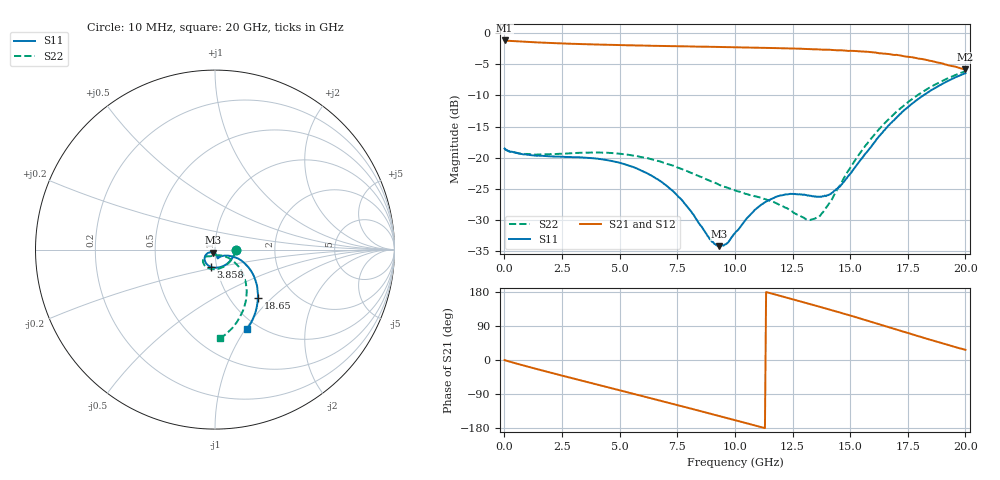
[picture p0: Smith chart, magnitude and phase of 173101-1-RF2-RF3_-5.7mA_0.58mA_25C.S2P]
!  2-Port S-parameters saved by WinCal
! VAR MeasName=S-Parameters (CALIBRATED_DATA) read from VNA (N5242A)
! VAR MeasDate=2017-7-20 9:31:15
! VAR NAME=173101-1-RF2-RF3_-5.7mA_0.58mA_25C
! VAR FILENAME=173101-1-RF2-RF3_-5.7mA_0.58mA_25C.S2P
! VAR DATE=2017-7-20 9:31:15
! VAR PHYS_PORTS=1,2
# Hz S DB R 50
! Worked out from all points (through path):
!   401 points, 10 MHz to 20 GHz, reference 50 ohm
!   highest |S21| = -1.18 dB at 10 MHz (marker M1); lowest = -5.8 dB at 20 GHz (marker M2)
!   group delay of S21, straight-line fit = 45.8 ps
!   lowest |S11| = -34.2 dB at 9.305 GHz (marker M3), VSWR 1.04, Z = 49.1 - j1.73 ohm
!   |S11| at or under -10 dB: start of sweep to 18.17 GHz
!   |S22| runs from -30.0 to -6.1 dB; largest |S21 - S12| = 0.0083
!   S11 on the Smith chart (normalised r, x): 10 MHz: 1.27, -0.00; 3.858 GHz: 0.94, -0.18; 18.65 GHz: 1.34, -0.83; 20 GHz: 0.89, -1.02
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1e7  -18.53 -0.9  -1.18 -0.2  -1.18 -0.3  -18.51 -1.2
1.559225e9  -19.67 -50.8  -1.51 -26.3  -1.51 -26.3  -19.46 -51.2
3.358325e9  -19.96 -92.9  -1.77 -54.5  -1.77 -54.5  -19.20 -91.2
3.858075e9  -20.09 -102.7  -1.82 -62.3  -1.82 -62.2  -19.16 -99.8
5.357325e9  -21.21 -128.6  -1.95 -85.5  -1.97 -85.4  -19.52 -121.7
6.70665e9  -23.60 -146.8  -2.05 -106.6  -2.04 -106.4  -20.54 -135.8
7.70615e9  -26.81 -154.0  -2.12 -122.1  -2.14 -122.0  -21.82 -141.9
8.90555e9  -33.03 -136.4  -2.19 -141.1  -2.20 -140.9  -23.68 -142.8
9.30535e9  -34.19 -115.6  -2.22 -147.5  -2.22 -147.4  -24.32 -141.4
9.6052e9  -33.89 -98.9  -2.24 -152.3  -2.24 -152.1  -24.72 -140.1
1.0005e10  -32.09 -83.0  -2.27 -158.7  -2.28 -158.6  -25.23 -137.2
1.085458e10  -28.40 -70.7  -2.33 -172.4  -2.34 -172.3  -26.17 -130.4
1.145428e10  -26.81 -71.0  -2.38 177.8  -2.38 177.9  -26.81 -125.2
1.230385e10  -25.87 -73.1  -2.45 163.6  -2.46 163.8  -28.20 -114.5
1.335332e10  -26.19 -65.9  -2.58 146.0  -2.57 146.2  -29.88 -81.0
1.375312e10  -26.28 -57.3  -2.64 139.0  -2.64 139.3  -29.01 -61.8
1.455272e10  -24.67 -35.4  -2.74 125.4  -2.74 125.6  -24.47 -36.4
1.575212e10  -18.97 -21.4  -3.01 103.5  -3.02 103.8  -17.67 -33.3
1.670165e10  -14.72 -25.1  -3.37 86.1  -3.42 86.2  -13.72 -41.1
1.76012e10  -11.59 -34.6  -3.83 69.7  -3.83 70.0  -10.82 -52.2
1.865068e10  -8.88 -48.4  -4.58 50.0  -4.64 50.6  -8.33 -66.9
2e10  -6.44 -67.8  -5.83 26.9  -5.88 27.6  -6.11 -86.5
